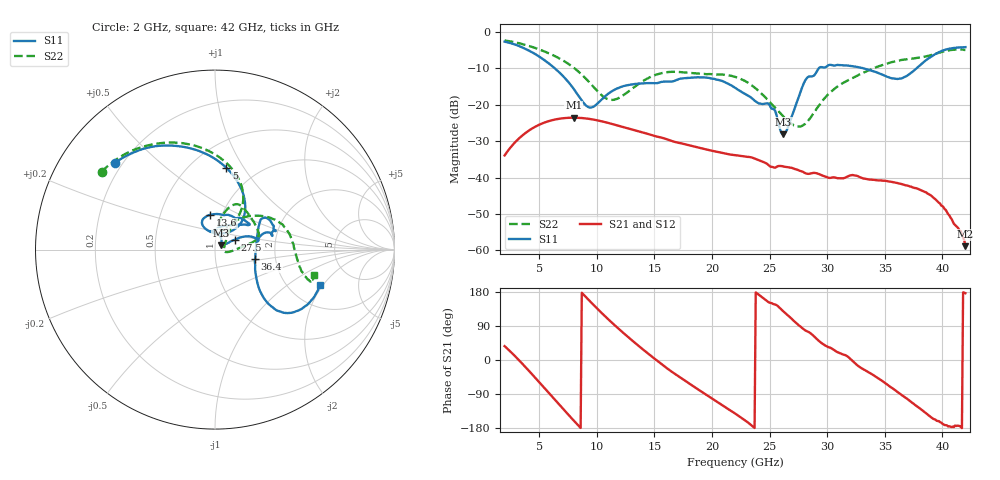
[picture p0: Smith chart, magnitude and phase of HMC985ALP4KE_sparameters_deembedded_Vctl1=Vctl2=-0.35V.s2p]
!s2p File: Measurements: S11, S21, S12, S22
# GHz S dB R 50.0
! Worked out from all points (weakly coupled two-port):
!   401 points, 2 GHz to 42 GHz, reference 50 ohm
!   highest |S21| = -23.54 dB at 8 GHz (marker M1); lowest = -58.9 dB at 42 GHz (marker M2)
!   lowest |S11| = -28.1 dB at 26.2 GHz (marker M3), VSWR 1.08, Z = 53.2 + j2.44 ohm
!   |S11| at or under -10 dB: 6.366 GHz to 29.27 GHz (22.9 GHz wide, 129 % of centre); 33.18 GHz to 37.75 GHz (4.569 GHz wide, 12.9 % of centre)
!   |S22| runs from -26.0 to -2.3 dB; largest |S21 - S12| = 0.00016
!   S11 on the Smith chart (normalised r, x): 2 GHz: 0.17, +0.36; 5 GHz: 0.73, +0.84; 13.6 GHz: 0.88, +0.35; 27.5 GHz: 1.24, +0.14; 36.4 GHz: 1.56, -0.17; 42 GHz: 2.93, -1.90
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2  -2.64 139.1  -33.92 36.6  -33.94 36.6  -2.31 145.5
3.4  -4.04 112.6  -28.82 -5.4  -28.82 -5.4  -3.19 123.2
5  -6.74 82.2  -25.48 -58.5  -25.49 -58.5  -4.76 98.7
8  -15.64 45.7  -23.54 -159.9  -23.54 -159.8  -9.79 60.9
8.7  -18.84 55.3  -23.64 177.4  -23.64 177.4  -11.71 56.2
9.6  -20.68 89.8  -24.00 149.1  -24.00 149.1  -14.66 54.8
11.1  -16.71 117.0  -25.07 104.5  -25.08 104.5  -18.60 69.6
13.6  -14.19 98.5  -27.26 38.1  -27.27 38.1  -14.33 78.0
15.4  -13.91 73.5  -28.85 -5.2  -28.86 -5.2  -11.48 68.3
19.4  -12.51 35.8  -32.20 -89.8  -32.19 -89.8  -11.54 34.7
22  -15.29 53.3  -33.84 -141.0  -33.84 -140.9  -12.32 14.3
25  -20.06 94.3  -36.84 151.3  -36.84 151.3  -19.19 -1.0
26.2  -28.13 35.7  -36.95 128.2  -36.95 128.3  -23.20 -11.8
27.5  -18.11 26.6  -37.98 92.6  -38.00 92.7  -25.99 -0.3
28.1  -13.29 19.4  -38.79 78.0  -38.79 78.2  -25.23 19.3
28.7  -12.18 11.8  -38.77 67.1  -38.80 67.2  -22.87 35.7
31.1  -9.11 23.1  -40.21 18.2  -40.21 18.1  -14.54 54.5
33.3  -10.10 33.5  -40.36 -27.0  -40.38 -27.0  -10.98 41.7
35.4  -12.49 11.9  -41.12 -69.2  -41.13 -68.9  -8.48 25.6
36.4  -12.79 -13.3  -41.74 -90.7  -41.77 -90.8  -7.70 17.0
39.6  -5.72 -42.8  -46.62 -161.0  -46.70 -161.4  -5.79 -15.7
42  -4.15 -18.7  -58.87 176.3  -58.59 178.0  -4.92 -14.5
